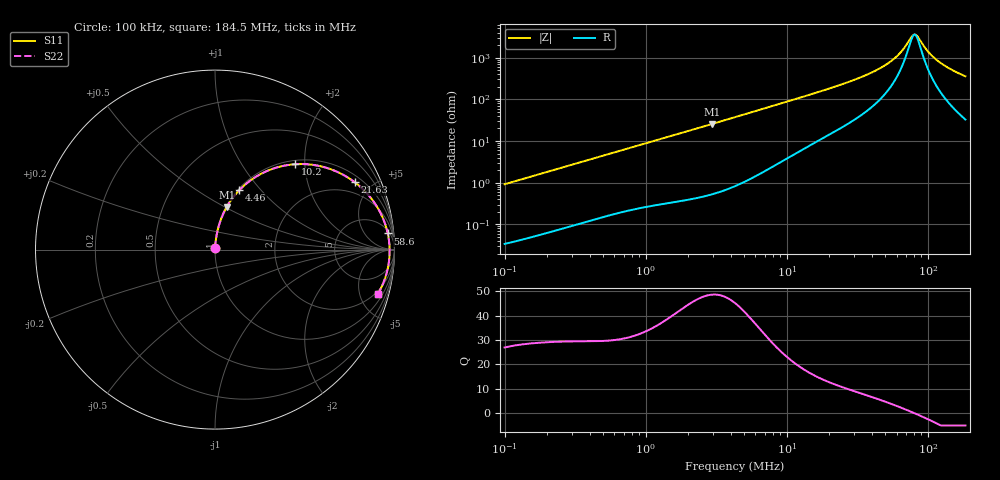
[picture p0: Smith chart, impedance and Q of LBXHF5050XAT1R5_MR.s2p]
! LBXHF5050XAT1R5_MR  S-PARAMETER MODEL  ( General Type )
! Model Generated by TAIYO YUDEN Corporation (http://www.ty-top.com)
! Version 2.0
! TAIYO YUDEN Control No. 201118NI43SB-FBB
! Copyright(c) 2020 TAIYO YUDEN CO.,LTD. All Rights Reserved.
! Product Description (link to TY-COMPAS)
! https://ds.yuden.co.jp/TYCOMPAS/or/detail?pn=LBXHF5050XAT1R5NMR&u=M
! Products Name : Inductors
! Characteristics :
!  Inductance : 1.5 uH , SRF(min) : 60 MHz , DC Resistance(max) : 0.0216 Ohm
!  Rated Current : Saturation :6300 mA , Temp Rise : 2800 mA
!  Case Size : 5.0 x 5.0 / 0.197 x 0.197 [mm/inch] , Thickness : 3.1 / 0.122 [mm/inch]
!  (Conditions: Temperature = 25 degC , DC Bias Current/Voltage = 0A / 0V)
! External Node Assignments :
!  1  o---GGG---o  2
! GND o---------o GND
! Frequency Range : 0.1MHz  -  184.468258MHz  [ 402 STEP ]
# MHz S RI R 50
! Freq[MHz].  S11 Real  S11 Imag  S21 Real  S21 Imag  S12 Real  S12 Imag  S22 Real  S22 Imag
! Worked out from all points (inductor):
!   401 points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, 100 kHz to 184.5 MHz, reference 50 ohm
!   read as one part in series: L = 1.46 uH near 103.8 kHz
!   highest Q = 48.6 at 2.949 MHz (marker M1), where L = 1.38 uH
!   self-resonance near 80.54 MHz
!   S11 on the Smith chart (normalised r, x): 100 kHz: 1.00, +0.02; 4.46 MHz: 1.02, +0.78; 10.2 MHz: 1.08, +1.79; 21.63 MHz: 1.33, +3.95; 58.6 MHz: 7, +19; 184.5 MHz: 1.66, -7.11
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0.1  0.000425 0.00917  0.9996 -0.00917  0.9996 -0.00917  0.000425 0.00917
0.352405  0.00207 0.0316  0.9979 -0.0316  0.9979 -0.0316  0.00207 0.0316
1.241892  0.0145 0.1065  0.9855 -0.1065  0.9855 -0.1065  0.0145 0.1065
2.948932  0.0658 0.2378  0.9342 -0.2378  0.9342 -0.2378  0.0658 0.2378
4.294977  0.1277 0.3229  0.8723 -0.3229  0.8723 -0.3229  0.1277 0.3229
4.459544  0.1362 0.3319  0.8638 -0.3319  0.8638 -0.3319  0.1362 0.3319
6.618374  0.2564 0.4221  0.7436 -0.4221  0.7436 -0.4221  0.2564 0.4221
10.19863  0.4476 0.4757  0.5524 -0.4757  0.5524 -0.4757  0.4476 0.4757
15.13571  0.6364 0.4507  0.3636 -0.4507  0.3636 -0.4507  0.6364 0.4507
21.63386  0.7781 0.3758  0.2219 -0.3758  0.2219 -0.3758  0.7781 0.3758
36.62254  0.9098 0.2269  0.0902 -0.2269  0.0902 -0.2269  0.9098 0.2269
45.03616  0.9393 0.1662  0.0607 -0.1662  0.0607 -0.1662  0.9393 0.1662
53.33896  0.9559 0.1172  0.0441 -0.1172  0.0441 -0.1172  0.9559 0.1172
58.59608  0.9626 0.0903  0.0374 -0.0903  0.0374 -0.0903  0.9626 0.0903
66.83781  0.969 0.0529  0.031 -0.0529  0.031 -0.0529  0.969 0.0529
76.23877  0.9724 0.0156  0.0276 -0.0156  0.0276 -0.0156  0.9724 0.0156
80.66224  0.9729 -0.000419  0.0271 0.000419  0.0271 0.000419  0.9729 -0.000419
85.34237  0.9729 -0.0164  0.0271 0.0164  0.0271 0.0164  0.9729 -0.0164
99.19348  0.9701 -0.0595  0.0299 0.0595  0.0299 0.0595  0.9701 -0.0595
115.2926  0.9631 -0.1033  0.0369 0.1033  0.0369 0.1033  0.9631 -0.1033
141.7798  0.9457 -0.1653  0.0543 0.1653  0.0543 0.1653  0.9457 -0.1653
184.4683  0.9078 -0.2469  0.0922 0.2469  0.0922 0.2469  0.9078 -0.2469
